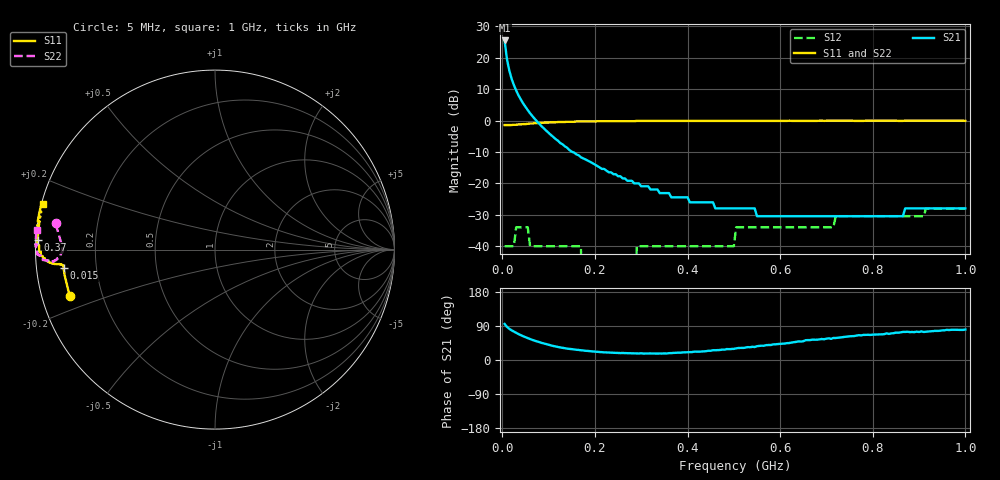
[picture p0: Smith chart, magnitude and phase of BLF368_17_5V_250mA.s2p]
! Filename:  BLF368_17.5V_250mA.s2p
! Philips part #: BLF368  !date: 21-05-2003
!17.5V @250 mA
!D:\Vee measurements\measurement data\VDMOST\BLF368\17.5V_250mA_#1
# HZ S MA R 50
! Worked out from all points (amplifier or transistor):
!   200 points, 5 MHz to 1 GHz, reference 50 ohm
!   highest |S21| = 25.5 dB at 5 MHz (marker M1)
!   |S21| within 3 dB of that: start of sweep to 7.532 MHz
!   S11 on the Smith chart (normalised r, x): 5 MHz: 0.08, -0.15; 15 MHz: 0.08, -0.06; 370 MHz: 0.01, +0.03; 1 GHz: 0.01, +0.13
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5000000  0.85 -162.3  18.93 95.2  0.01 2.7  0.9 170.7
1e7  0.85 -170.5  9.57 87.5  0.01 21.8  0.87 175.2
1.5e7  0.85 -173.0  6.33 82.4  0.01 22.4  0.86 177.1
2e7  0.85 -174.1  4.67 78.4  0.01 18.5  0.85 178.4
2.5e7  0.86 -174.4  3.69 75.0  0.01 13.6  0.85 179.5
3e7  0.86 -174.6  3.02 71.5  0.02 8.4  0.85 -179.9
4e7  0.87 -174.7  2.17 65.5  0.02 -0.1  0.86 -178.3
5.5e7  0.89 -174.8  1.47 57.7  0.02 -10.2  0.88 -176.8
6e7  0.9 -174.9  1.31 55.3  0.01 -13.0  0.88 -176.5
9.5e7  0.93 -175.8  0.69 41.7  0.01 -25.9  0.92 -175.8
1.7e8  0.97 -178.3  0.26 25.7  0.01 -22.6  0.96 -176.7
1.75e8  0.97 -178.5  0.25 25.1  0 -20.6  0.97 -176.8
2.85e8  0.98 178.6  0.1 17.5  0 67.2  0.99 -178.8
2.9e8  0.99 178.5  0.1 17.3  0.01 68.9  0.99 -178.9
3.4e8  0.99 177.5  0.07 17.1  0.01 76.2  0.99 -179.5
3.7e8  0.99 176.9  0.06 18.7  0.01 81.4  0.99 -179.9
5e8  0.99 174.3  0.04 29.4  0.01 88.3  1 178.6
5.05e8  0.99 174.3  0.04 30.7  0.02 88.2  1 178.5
6.7e8  0.99 171.3  0.03 53.8  0.02 90.5  1 176.9
7.2e8  1 170.4  0.03 58.0  0.03 90.9  1 176.5
8.35e8  1 168.3  0.03 68.8  0.03 92.8  1 175.4
1e9  0.99 165.1  0.04 80.4  0.04 91.8  1 173.7
